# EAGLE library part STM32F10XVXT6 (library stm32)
STM32F101/103 100 pin LQFP
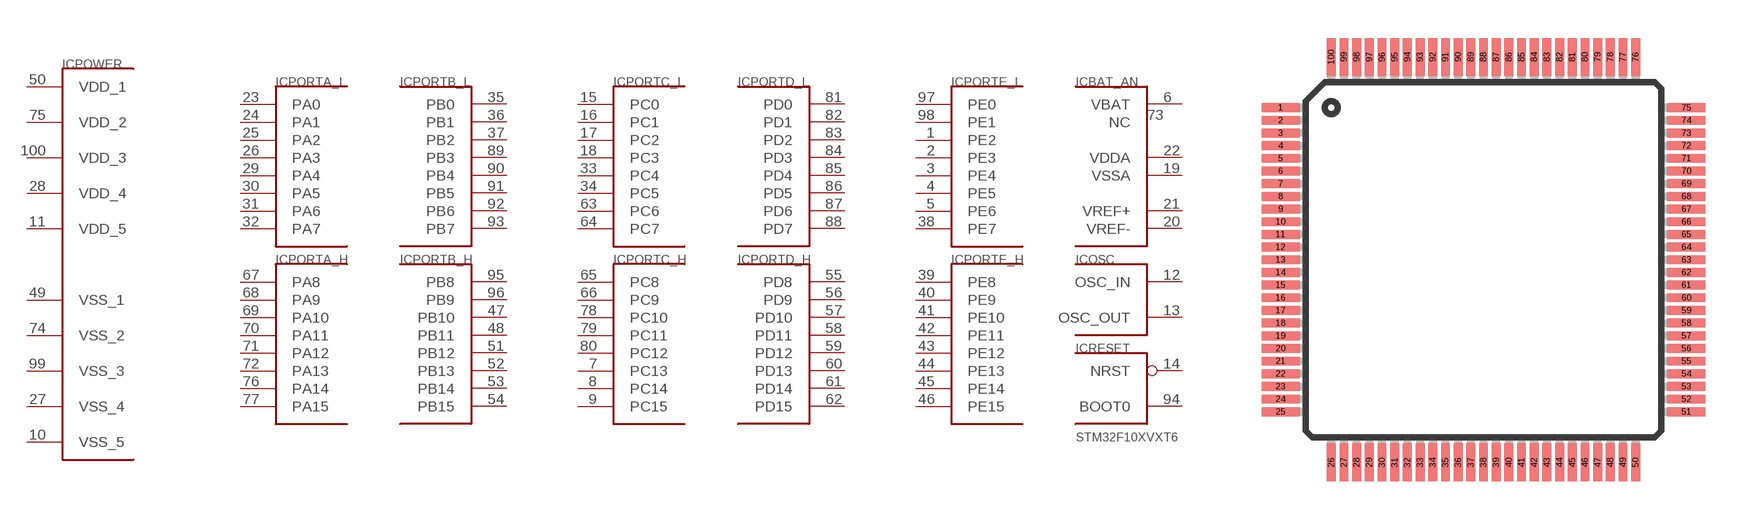
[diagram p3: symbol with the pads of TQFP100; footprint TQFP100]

Designator prefix IC; gates PORTA_L=PORT_A_L PORTA_H=PORT_A_H PORTB_L=PORT_B_L PORTB_H=PORT_B_H PORTC_L=PORT_C_L PORTC_H=PORT_C_H PORTD_L=PORT_D_L PORTD_H=PORT_D_H PORTE_L=PORT_E_L PORTE_H=PORT_E_H POWER=VCC_VSS_L BAT_AN=BAT_AN_L OSC=OSC RESET=BOOT_RST

## STM32F10XVXT6  [TQFP100]
1  PORTE_L:PE2
2  PORTE_L:PE3
3  PORTE_L:PE4
4  PORTE_L:PE5
5  PORTE_L:PE6
6  BAT_AN:VBAT  pwr
7  PORTC_H:PC13
8  PORTC_H:PC14
9  PORTC_H:PC15
10  POWER:VSS_5  pwr
11  POWER:VDD_5  pwr
12  OSC:OSC_IN  in
13  OSC:OSC_OUT  out
14  RESET:NRST  in
15  PORTC_L:PC0
16  PORTC_L:PC1
17  PORTC_L:PC2
18  PORTC_L:PC3
19  BAT_AN:VSSA  pwr
20  BAT_AN:VREF-  in
21  BAT_AN:VREF+  in
22  BAT_AN:VDDA  pwr
23  PORTA_L:PA0
24  PORTA_L:PA1
25  PORTA_L:PA2
26  PORTA_L:PA3
27  POWER:VSS_4  pwr
28  POWER:VDD_4  pwr
29  PORTA_L:PA4
30  PORTA_L:PA5
31  PORTA_L:PA6
32  PORTA_L:PA7
33  PORTC_L:PC4
34  PORTC_L:PC5
35  PORTB_L:PB0
36  PORTB_L:PB1
37  PORTB_L:PB2
38  PORTE_L:PE7
39  PORTE_H:PE8
40  PORTE_H:PE9
41  PORTE_H:PE10
42  PORTE_H:PE11
43  PORTE_H:PE12
44  PORTE_H:PE13
45  PORTE_H:PE14
46  PORTE_H:PE15
47  PORTB_H:PB10
48  PORTB_H:PB11
49  POWER:VSS_1  pwr
50  POWER:VDD_1  pwr
51  PORTB_H:PB12
52  PORTB_H:PB13
53  PORTB_H:PB14
54  PORTB_H:PB15
55  PORTD_H:PD8
56  PORTD_H:PD9
57  PORTD_H:PD10
58  PORTD_H:PD11
59  PORTD_H:PD12
60  PORTD_H:PD13
61  PORTD_H:PD14
62  PORTD_H:PD15
63  PORTC_L:PC6
64  PORTC_L:PC7
65  PORTC_H:PC8
66  PORTC_H:PC9
67  PORTA_H:PA8
68  PORTA_H:PA9
69  PORTA_H:PA10
70  PORTA_H:PA11
71  PORTA_H:PA12
72  PORTA_H:PA13
73  BAT_AN:NC  nc
74  POWER:VSS_2  pwr
75  POWER:VDD_2  pwr
76  PORTA_H:PA14
77  PORTA_H:PA15
78  PORTC_H:PC10
79  PORTC_H:PC11
80  PORTC_H:PC12
81  PORTD_L:PD0
82  PORTD_L:PD1
83  PORTD_L:PD2
84  PORTD_L:PD3
85  PORTD_L:PD4
86  PORTD_L:PD5
87  PORTD_L:PD6
88  PORTD_L:PD7
89  PORTB_L:PB3
90  PORTB_L:PB4
91  PORTB_L:PB5
92  PORTB_L:PB6
93  PORTB_L:PB7
94  RESET:BOOT0  in
95  PORTB_H:PB8
96  PORTB_H:PB9
97  PORTE_L:PE0
98  PORTE_L:PE1
99  POWER:VSS_3  pwr
100  POWER:VDD_3  pwr

## Footprint TQFP100 (pad centres in mm)
smd 1.5 x 0.35: 1 -8,6; 2 -8,5.5; 3 -8,5; 4 -8,4.5; 5 -8,4; 6 -8,3.5; 7 -8,3; 8 -8,2.5; 9 -8,2; 10 -8,1.5; 11 -8,1; 12 -8,0.5; 13 -8,0; 14 -8,-0.5; 15 -8,-1; 16 -8,-1.5; 17 -8,-2; 18 -8,-2.5; 19 -8,-3; 20 -8,-3.5; 21 -8,-4; 22 -8,-4.5; 23 -8,-5; 24 -8,-5.5; 25 -8,-6; 51 8,-6; 52 8,-5.5; 53 8,-5; 54 8,-4.5; 55 8,-4; 56 8,-3.5; 57 8,-3; 58 8,-2.5; 59 8,-2; 60 8,-1.5; 61 8,-1; 62 8,-0.5; 63 8,0; 64 8,0.5; 65 8,1; 66 8,1.5; 67 8,2; 68 8,2.5; 69 8,3; 70 8,3.5; 71 8,4; 72 8,4.5; 73 8,5; 74 8,5.5; 75 8,6
smd 0.35 x 1.5: 26 -6,-8; 27 -5.5,-8; 28 -5,-8; 29 -4.5,-8; 30 -4,-8; 31 -3.5,-8; 32 -3,-8; 33 -2.5,-8; 34 -2,-8; 35 -1.5,-8; 36 -1,-8; 37 -0.5,-8; 38 0,-8; 39 0.5,-8; 40 1,-8; 41 1.5,-8; 42 2,-8; 43 2.5,-8; 44 3,-8; 45 3.5,-8; 46 4,-8; 47 4.5,-8; 48 5,-8; 49 5.5,-8; 50 6,-8; 76 6,8; 77 5.5,8; 78 5,8; 79 4.5,8; 80 4,8; 81 3.5,8; 82 3,8; 83 2.5,8; 84 2,8; 85 1.5,8; 86 1,8; 87 0.5,8; 88 0,8; 89 -0.5,8; 90 -1,8; 91 -1.5,8; 92 -2,8; 93 -2.5,8; 94 -3,8; 95 -3.5,8; 96 -4,8; 97 -4.5,8; 98 -5,8; 99 -5.5,8; 100 -6,8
